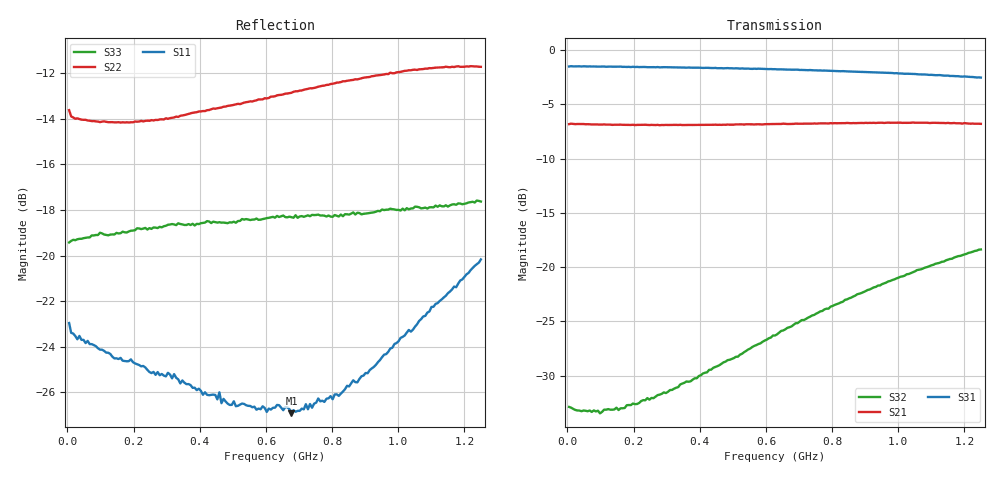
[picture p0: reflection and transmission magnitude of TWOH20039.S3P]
!Agilent Technologies,E5071B,MY42403515,A.09.10
!Date: Mon Feb 19 09:38:41 2024
!Data & Calibration Information:
!Freq	S11:SOLT3(ON)	S12:SOLT3(ON)	S13:SOLT3(ON)
!	S21:SOLT3(ON)	S22:SOLT3(ON)	S23:SOLT3(ON)
!	S31:SOLT3(ON)	S32:SOLT3(ON)	S33:SOLT3(ON)
# Hz S dB R 50
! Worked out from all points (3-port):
!   201 points, 5 MHz to 1.25 GHz, reference 50 ohm
!   strongest paths, dB at 5 MHz, 316.2 MHz, 627.5 MHz, 938.8 MHz, 1.25 GHz:
!     S31: -1.5, -1.6, -1.8, -2.1, -2.5
!     S21: -6.8, -6.9, -6.8, -6.7, -6.8
!     S32: -32.9, -31.3, -26.3, -21.7, -18.4
!   lowest |S11| = -26.9 dB at 677.3 MHz (marker M1), VSWR 1.09, Z = 52.4 + j3.94 ohm
!   |S11| at or under -10 dB: start of sweep to end of sweep
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5000000  -22.96 167.3  -6.80 -179.8  -1.50 0.2
         -6.83 -179.8  -13.62 170.2  -32.95 30.1
         -1.52 0.2  -32.89 29.7  -19.42 12.2
2.99e7  -23.67 171.5  -6.81 175.8  -1.50 -2.5
        -6.82 175.9  -13.98 170.8  -33.22 6.7
        -1.51 -2.6  -33.22 6.1  -19.28 1.4
1.544e8  -24.53 152.4  -6.86 159.2  -1.54 -13.4
         -6.88 159.1  -14.15 142.9  -33.21 13.9
         -1.53 -13.3  -33.17 13.3  -19.03 -6.2
3.47375e8  -25.47 120.5  -6.89 133.8  -1.62 -30.0
           -6.91 133.8  -13.85 100.3  -30.75 30.4
           -1.61 -29.9  -30.74 30.5  -18.63 -18.4
4.84325e8  -26.49 95.6  -6.87 116.1  -1.68 -41.8
           -6.86 116.1  -13.43 72.4  -28.55 34.2
           -1.66 -41.8  -28.58 34.5  -18.57 -26.7
6.275e8  -26.67 68.5  -6.83 98.0  -1.78 -54.3
         -6.82 97.8  -13.01 43.7  -26.30 34.6
         -1.76 -54.3  -26.31 34.6  -18.33 -35.1
6.773e8  -26.91 56.3  -6.80 91.5  -1.80 -58.6
         -6.79 91.5  -12.86 33.8  -25.45 33.5
         -1.81 -58.6  -25.47 33.5  -18.32 -37.8
8.20475e8  -26.15 25.6  -6.75 73.6  -1.96 -71.0
           -6.74 73.6  -12.40 6.4  -23.35 27.8
           -1.94 -71.1  -23.35 27.5  -18.28 -45.8
9.761e8  -24.07 -3.6  -6.68 54.3  -2.11 -84.9
         -6.70 54.2  -11.97 -22.7  -21.28 19.2
         -2.11 -84.8  -21.28 19.3  -17.94 -53.0
1.25e9  -20.16 -45.7  -6.81 19.8  -2.52 -109.7
        -6.80 19.9  -11.72 -73.6  -18.36 -0.8
        -2.53 -109.7  -18.38 -0.9  -17.63 -64.0
